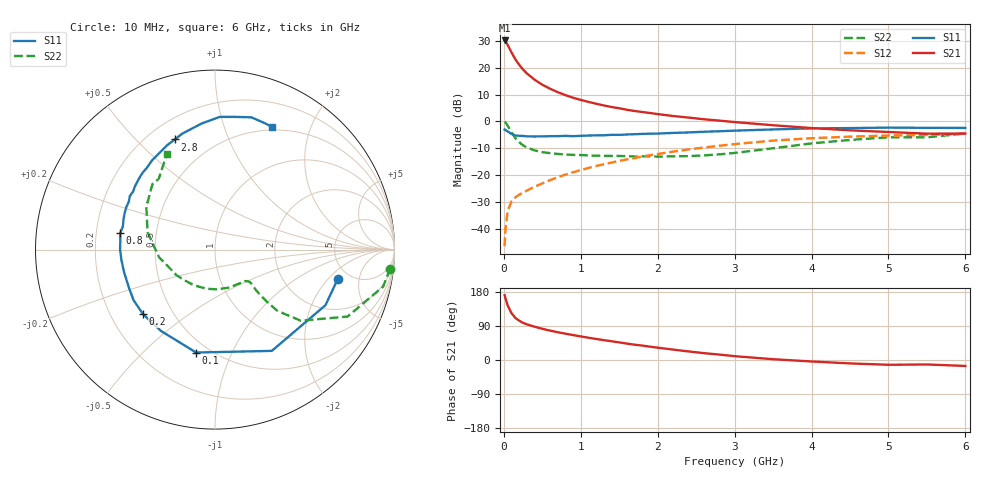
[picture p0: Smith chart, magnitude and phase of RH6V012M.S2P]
! SIEMENS Small Signal Semiconductors
! BFR106
! Si NPN RF Bipolar Junction Transistor in SOT23
! VCE = 6 V  IC = 12 mA
! Common Emitter S-Parameters:  August  1996
# GHz  S  MA  R  50
!  f  S11  S21  S12  S22
! GHz  MAG  ANG  MAG  ANG  MAG  ANG  MAG  ANG
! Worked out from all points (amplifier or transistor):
!   36 points, 10 MHz to 6 GHz, reference 50 ohm
!   highest |S21| = 30.2 dB at 10 MHz (marker M1)
!   |S21| within 3 dB of that: start of sweep to 73.42 MHz
!   unconditionally stable (mu >= 1): 459 MHz to 2.044 GHz; 5.428 GHz to end of sweep
!   at 250 MHz: K = 0.76, MSG = 23.0 dB, |S12| = -26.6 dB
!   at 1.4 GHz: K = 1.08, MAG = 8.7 dB, |S12| = -15.4 dB
!   at 6 GHz: K = 1.00, MAG = -0.3 dB, |S12| = -4.6 dB
!   S11 on the Smith chart (normalised r, x): 10 MHz: 4.00, -2.58; 100 MHz: 0.43, -0.74; 200 MHz: 0.34, -0.34; 800 MHz: 0.30, +0.08; 2.8 GHz: 0.31, +0.65; 6 GHz: 0.47, +1.47
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0.01  0.7034 -13.4  32.27 171.1  0.0047 85.7  0.9818 -6.2
0.02  0.6891 -26.7  31.39 163.8  0.0095 76.3  0.9591 -12.4
0.05  0.647 -60.7  26.52 143.9  0.0214 63.8  0.8276 -26.8
0.1  0.583 -100.4  19.29 123.5  0.0323 53.4  0.62 -39.7
0.15  0.544 -123.6  14.31 111.0  0.0383 49.2  0.4867 -44.5
0.2  0.5385 -138.3  11.35 103.7  0.0428 49.0  0.4102 -45.1
0.25  0.5341 -148.2  9.26 98.0  0.0468 50.6  0.3566 -45.0
0.3  0.5251 -155.5  7.822 94.1  0.0512 52.7  0.3262 -44.8
0.4  0.5223 -166.4  5.982 87.8  0.0605 55.8  0.2872 -43.5
0.5  0.5247 -174.0  4.819 82.3  0.0696 58.8  0.266 -42.9
0.6  0.529 179.9  4.063 77.6  0.0799 60.9  0.2554 -43.7
0.7  0.5302 174.2  3.509 73.3  0.0909 62.4  0.2472 -45.4
0.8  0.5359 170.2  3.083 69.5  0.1014 62.9  0.2403 -46.9
0.9  0.5293 165.8  2.756 65.8  0.1124 63.6  0.2372 -48.6
1.1  0.5436 157.5  2.306 58.8  0.1349 63.9  0.232 -54.9
1.6  0.5684 141.8  1.644 43.3  0.1953 61.7  0.2236 -72.7
2.2  0.6084 125.2  1.258 27.5  0.2725 55.9  0.2227 -100.9
2.8  0.6533 110.1  1.033 14.3  0.3505 47.8  0.2422 -135.9
3.5  0.7066 96.0  0.846 2.1  0.4372 36.9  0.3149 -172.3
4.5  0.7492 80.6  0.68 -9.0  0.5183 19.7  0.4503 148.2
5.5  0.7571 68.7  0.59 -11.8  0.5551 8.0  0.5033 128.6
6  0.7537 64.9  0.592 -15.7  0.5899 0.2  0.5942 116.9
